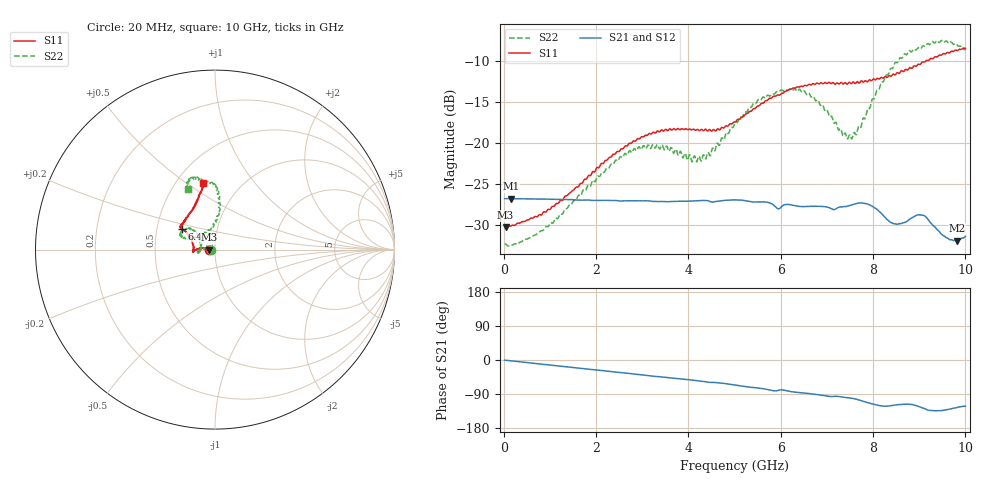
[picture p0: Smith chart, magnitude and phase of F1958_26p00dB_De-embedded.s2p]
! Integrated Device Technology
! Corporate Headquarters
! 6024 Silver Creek Valley Road
! San Jose, CA 95138  USA
! Phone:  1-408-284-8200
! Toll Free:  1-800-223-1366
! Webpage:  http://www.idt.com/
! Timing and RF Division
! 515 Groton Road, Suite 102
! Westford, MA 01886-6024
! Device:  F1958
! Description: 7-bit 0.25 dB Digital Step Attenuator
! Frequency:  0.001 -  6.000 GHz
! Package:  4x4 mm Thin QFN Plastic Package: 24 pin
! Ports:  2 RF, 12 DC
!  Pin  1  = D0
!  Pin  2  = VDD
!  Pin  3  = VMODE
!  Pin  4  = GND
!  Pin  5  = RF1  =  Port 1
!  Pin  6  = GND
!  Pin  7  = GND
!  Pin  8  = GND
!  Pin  9  = GND
!  Pin 10  = GND
!  Pin 11  = GND
!  Pin 12  = GND
!  Pin 13  = GND
!  Pin 14  = RF2  =  Port 2
!  Pin 15  = GND
!  Pin 16  = LE
!  Pin 17  = CLK
!  Pin 18  = DATA
!  Pin 19  = D6
!  Pin 20  = D5
!  Pin 21  = D4
!  Pin 22  = D3
!  Pin 23  = D2
!  Pin 24  = D1
! State:  104
! Atten State:  26.00 dB
! Voltage:  +3.30 Volts
! Current:  0.258 mA
! Data:  The device was measured on a F1958 evaluation board which has
!  individual transmission lines to the RF pins.  Data was collected
!  using a calibrated network analyzer.  The evaluation board was
!  de-embedded using Automatic Fixture Removal (AFR).
!  The reference plane is the edge of the package pin.
! Misc:
!  Action Tracker AT0419
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# GHz S dB R 50
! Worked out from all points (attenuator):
!   500 points, 20 MHz to 10 GHz, reference 50 ohm
!   highest |S21| = -26.75 dB at 160 MHz (marker M1); lowest = -31.9 dB at 9.82 GHz (marker M2)
!   lowest |S11| = -30.2 dB at 40 MHz (marker M3), VSWR 1.06, Z = 47 - j0.0416 ohm
!   |S11| at or under -10 dB: start of sweep to 9.139 GHz
!   |S22| runs from -32.5 to -7.5 dB; largest |S21 - S12| = 0.00034
!   S11 on the Smith chart (normalised r, x): 20 MHz: 0.94, -0.00; 6.4 GHz: 0.67, +0.16; 10 GHz: 0.67, +0.59
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0.02  -30.19 -179.0  -26.76 -0.3  -26.76 -0.2  -32.30 -178.9
0.04  -30.22 -179.2  -26.75 -0.5  -26.75 -0.5  -32.28 -178.4
0.16  -30.06 177.6  -26.75 -2.2  -26.75 -2.2  -32.34 178.1
0.84  -28.57 171.2  -26.80 -11.2  -26.80 -11.2  -30.66 172.3
1.7  -24.86 171.3  -26.93 -22.4  -26.92 -22.3  -25.98 171.5
2.62  -20.40 177.3  -27.02 -34.2  -27.00 -34.3  -21.26 -179.2
3.36  -18.59 -175.4  -27.10 -44.1  -27.10 -44.2  -20.51 -169.0
4.24  -18.48 -178.7  -27.00 -55.2  -27.01 -55.3  -21.63 169.3
4.5  -18.54 175.4  -27.16 -59.2  -27.17 -59.3  -21.01 151.7
5.02  -17.40 161.0  -26.90 -66.2  -26.91 -66.2  -17.42 138.4
5.58  -15.15 150.7  -27.15 -75.0  -27.16 -75.1  -14.67 140.1
6.4  -13.17 147.9  -27.68 -86.1  -27.70 -86.0  -13.42 155.9
6.68  -12.80 146.7  -27.68 -89.4  -27.69 -89.3  -14.34 158.0
7.5  -12.63 138.4  -27.59 -100.3  -27.59 -100.1  -18.96 120.3
7.68  -12.58 135.4  -27.29 -104.9  -27.28 -104.9  -18.02 100.1
7.9  -12.39 129.0  -27.45 -112.9  -27.44 -113.0  -15.73 89.6
8.34  -11.78 119.0  -29.45 -121.5  -29.45 -121.6  -11.51 84.1
8.66  -11.29 113.3  -29.69 -116.8  -29.72 -116.8  -9.29 87.8
9.08  -10.08 107.2  -28.77 -126.8  -28.78 -126.6  -8.12 98.9
9.54  -9.09 102.0  -31.29 -132.6  -31.31 -132.5  -7.70 108.9
9.82  -8.72 100.5  -31.85 -125.2  -31.87 -125.2  -8.04 113.4
10  -8.46 99.8  -31.36 -121.9  -31.38 -121.8  -8.64 113.9
